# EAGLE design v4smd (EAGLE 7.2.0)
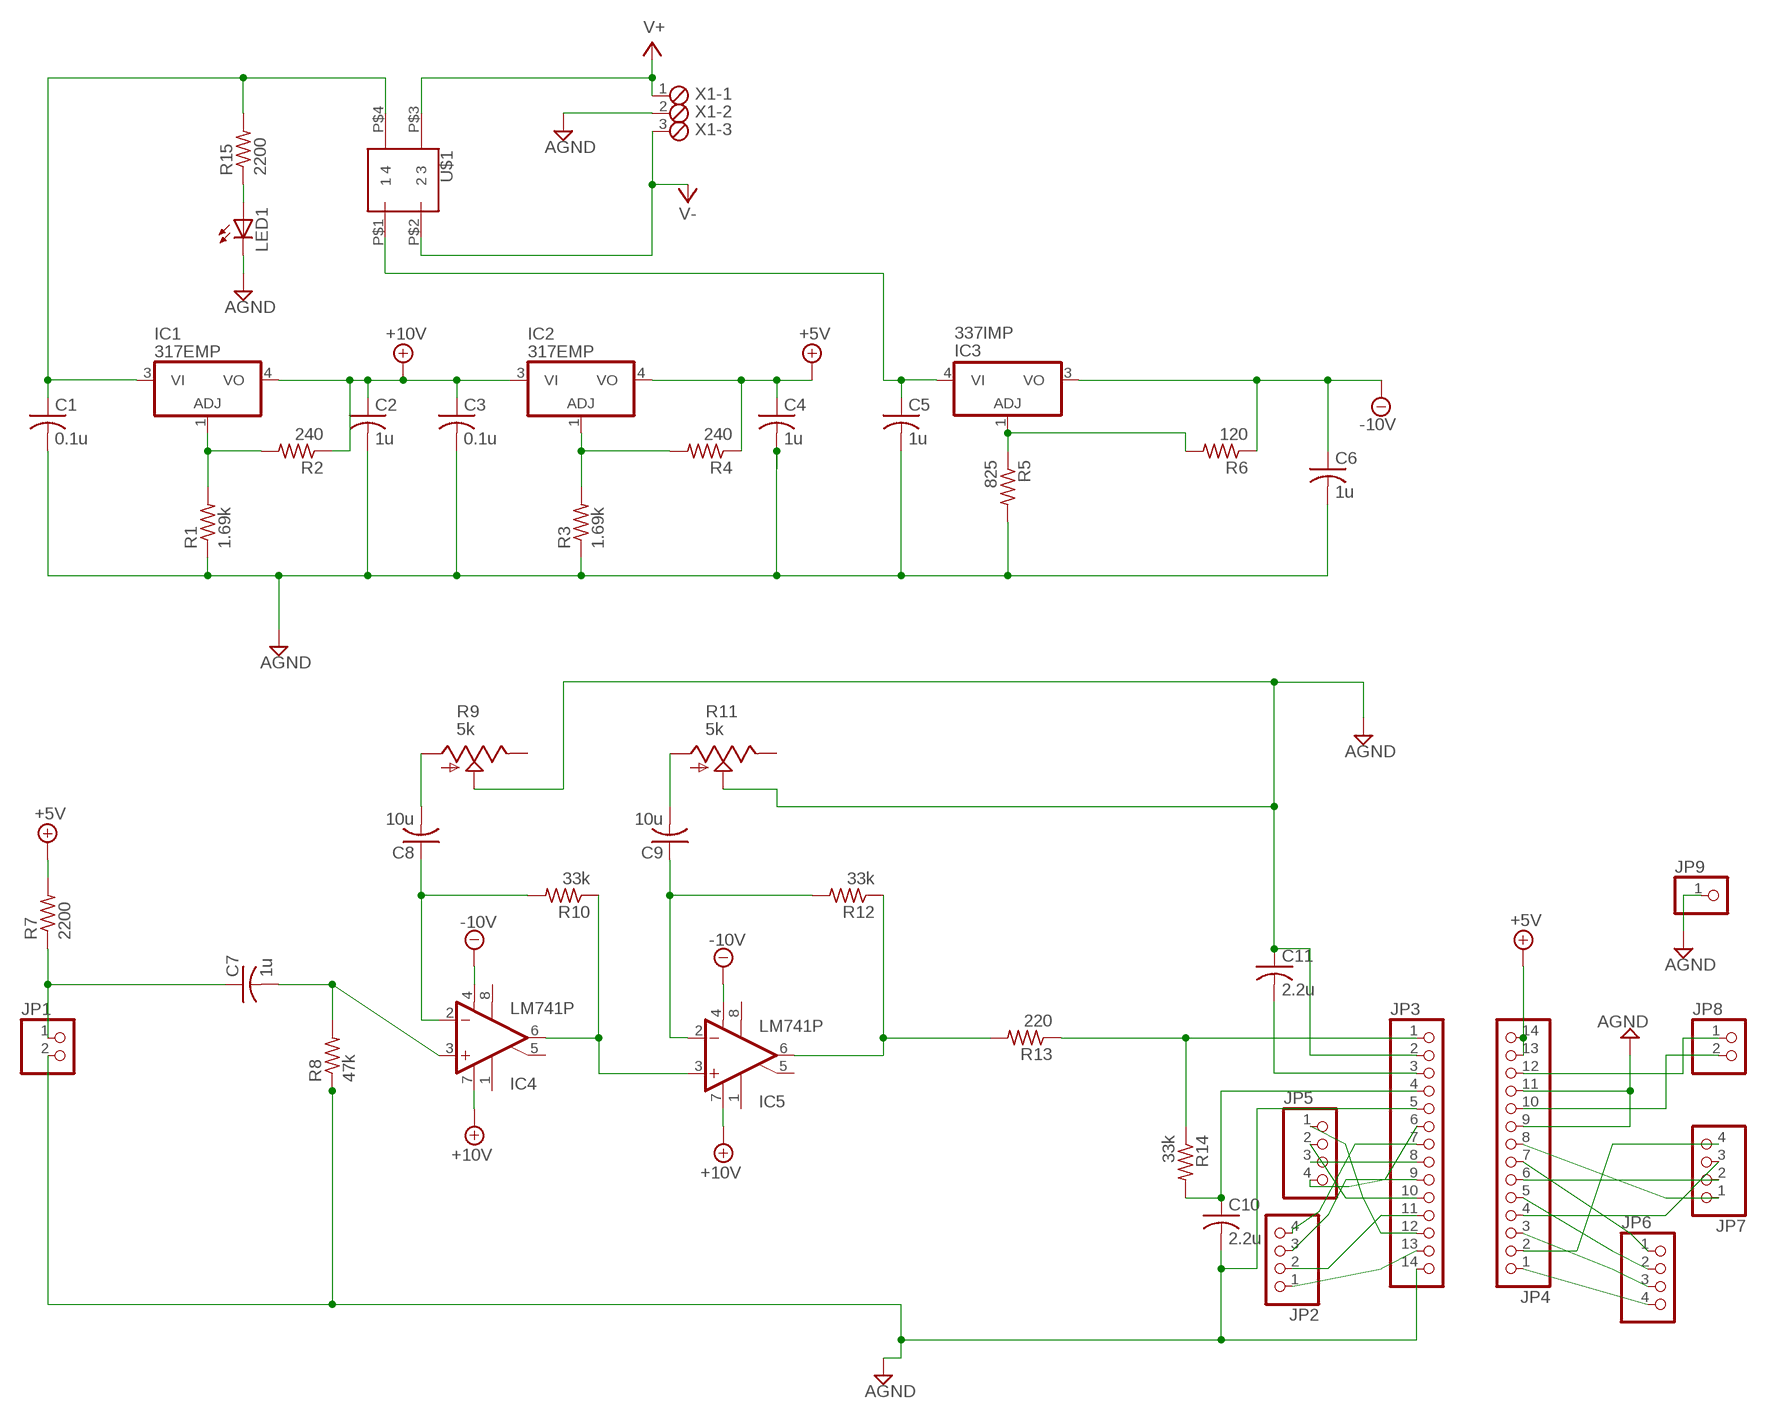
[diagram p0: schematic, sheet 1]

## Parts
C1  0.1u  C-USC1206  [C1206]
C2  1u  C-USC1206  [C1206]
C3  0.1u  C-USC1206  [C1206]
C4  1u  C-USC1206  [C1206]
C5  1u  C-USC1206  [C1206]
C6  1u  C-USC1206  [C1206]
C7  1u  C-USC1206  [C1206]
C8  10u  C-USC1206  [C1206]
C9  10u  C-USC1206  [C1206]
C10  2.2u  C-USC1206  [C1206]
C11  2.2u  C-USC1206  [C1206]
IC1  317EMP  [SOT223]
IC2  317EMP  [SOT223]
IC3  337IMP  [SOT223]
IC4  LM741P  [DIL08]
IC5  LM741P  [DIL08]
JP1  PINHD-1X2  [1X02]
JP2  PINHD-1X4/90  [1X04/90]
JP3  PINHD-1X14  [1X14]
JP4  PINHD-1X14  [1X14]
JP5  PINHD-1X4/90  [1X04/90]
JP6  PINHD-1X4/90  [1X04/90]
JP7  PINHD-1X4/90  [1X04/90]
JP8  PINHD-1X2  [1X02]
JP9  PINHD-1X1  [1X01]
LED1  LED3MM  [LED3MM]
R1  1.69k  R-US_R2512  [R2512]
R2  240  R-US_R2512  [R2512]
R3  1.69k  R-US_R2512  [R2512]
R4  240  R-US_R2512  [R2512]
R5  825  R-US_R2512  [R2512]
R6  120  R-US_R2512  [R2512]
R7  2200  R-US_R2512  [R2512]
R8  47k  R-US_R2512  [R2512]
R9  5k  TRIM_US-B64Y  [B64Y]
R10  33k  R-US_R2512  [R2512]
R11  5k  TRIM_US-B64Y  [B64Y]
R12  33k  R-US_R2512  [R2512]
R13  220  R-US_R2512  [R2512]
R14  33k  R-US_R2512  [R2512]
R15  2200  R-US_R2512  [R2512]
U$1  S201031MS02Q  [DPST_FOOTPRINT]
X1  MPT3  [3POL254]

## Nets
+5V: C4.1 IC2.4(VO) JP4.13 JP4.14 R4.1 R7.2
+10V: C2.1 C3.1 IC1.4(VO) IC2.3(VI) IC4.7(V+) IC5.7(V+) R2.1
-10V: C6.1 IC3.3(VO) IC4.4(V-) IC5.4(V-) R6.1
AGND: C1.2 C2.2 C3.2 C4.2 C5.2 C6.2 C10.2 C11.1 JP1.2 JP3.2 JP3.5 JP3.14 JP4.9 JP4.11 JP9.1 LED1.K(C) R1.1 R3.1 R5.2 R8.1 R9.S R11.S X1.2
N$1: IC4.6(OUT) IC5.3(+IN) R10.1
N$2: C7.1 JP1.1 R7.1
N$3: C7.2 IC4.3(+IN) R8.2
N$4: C8.1 IC4.2(-IN) R10.2
N$5: IC5.6(OUT) R12.1 R13.2
N$6: C9.1 IC5.2(-IN) R12.2
N$7: JP3.1 R13.1 R14.1
N$8: IC1.1(ADJ) R1.2 R2.2
N$9: IC2.1(ADJ) R3.2 R4.2
N$10: IC3.1(ADJ) R5.1 R6.2
N$11: C8.2 R9.A
N$12: JP4.2 JP7.4
N$13: JP4.3 JP6.3
N$14: C9.2 R11.A
N$15: C11.2 JP3.3
N$16: C10.1 JP3.4 R14.2
N$17: JP4.4 JP7.3
N$18: JP4.5 JP6.2
N$19: JP3.10 JP5.2
N$20: JP2.2 JP3.11
N$21: JP3.12 JP5.1
N$22: JP2.1 JP3.13
N$23: JP4.1 JP6.4
N$24: JP4.6 JP7.2
N$25: JP4.7 JP6.1
N$26: JP4.8 JP7.1
N$27: JP2.3 JP3.9
N$28: JP3.8 JP5.3
N$29: JP2.4 JP3.7
N$30: JP3.6 JP5.4
N$31: JP4.12 JP8.1
N$32: JP4.10 JP8.2
N$43: C1.1 IC1.3(VI) R15.2 U$1.P$4
N$44: C5.1 IC3.4(VI) U$1.P$1
N$45: LED1.A R15.1
V+: U$1.P$3 X1.1
V-: U$1.P$2 X1.3
Unconnected: IC4.1(ON1) IC4.5(ON2) IC4.8(OPT) IC5.1(ON1) IC5.5(ON2) IC5.8(OPT) R9.E R11.E

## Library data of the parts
C1-C11 = rcl:C-US: CAPACITOR, American symbol
IC1 IC2 = linear:*317: Positive VOLTAGE REGULATOR
IC3 = linear:*337: Negative VOLTAGE REGULATOR
IC4 IC5 = linear:*741: OP AMP
JP1 JP8 = pinhead:PINHD-1X2: PIN HEADER
JP2 JP5-JP7 = pinhead:PINHD-1X4: PIN HEADER
JP3 JP4 = pinhead:PINHD-1X14: PIN HEADER
JP9 = pinhead:PINHD-1X1: PIN HEADER
LED1 = led:LED: LED
R1-R8 R10 R12-R15 = rcl:R-US_: RESISTOR, American symbol
R9 R11 = pot:TRIM_US-: POTENTIOMETER
U$1 = mylib:S201031MS02Q
X1 = con-phoenix-254:MPT3: PHOENIX CONNECTOR; OC_FARNELL: unknown; OC_NEWARK: unknown

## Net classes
0 default: clearance 0.205 mm

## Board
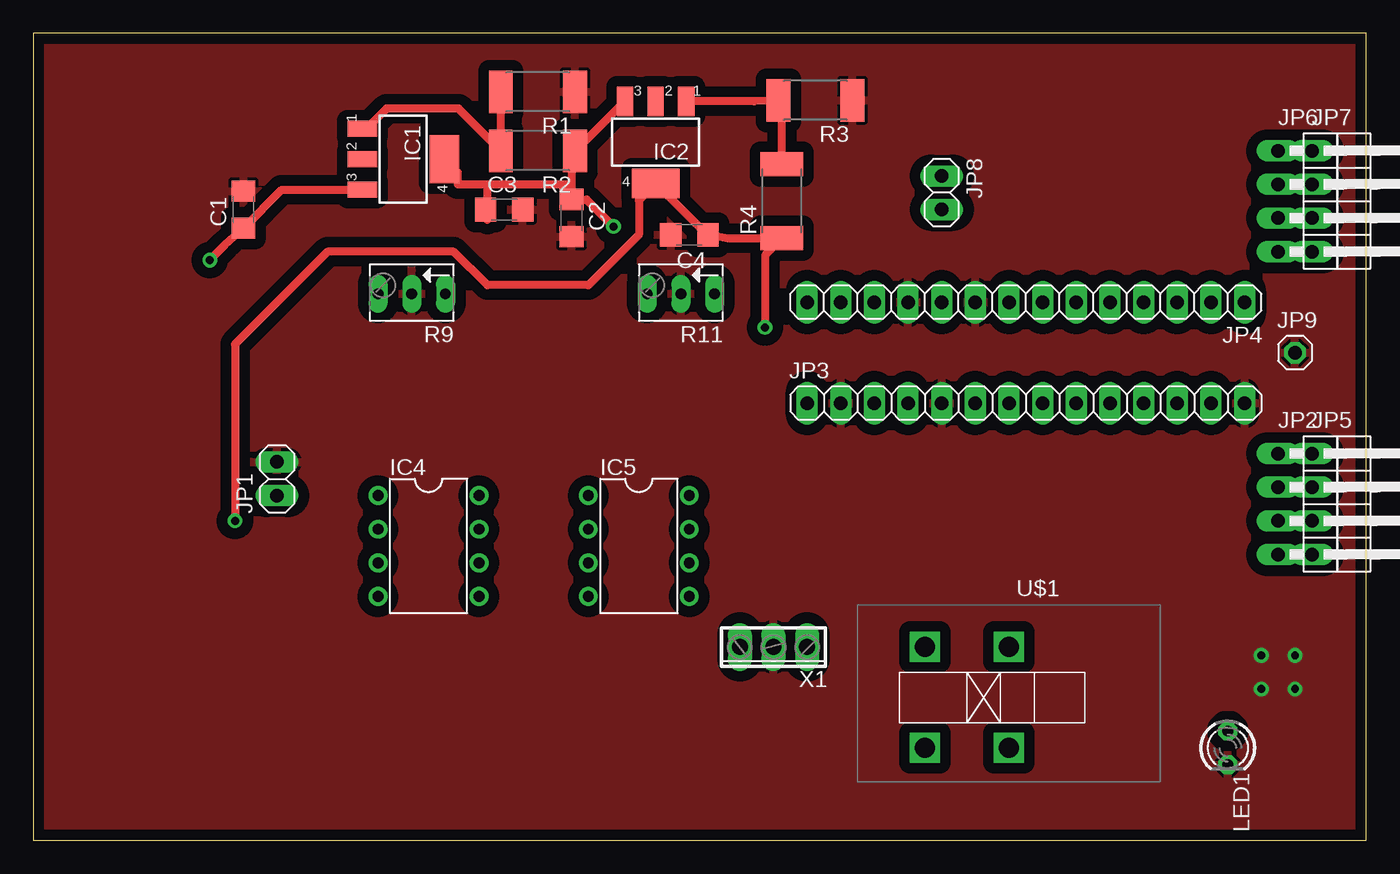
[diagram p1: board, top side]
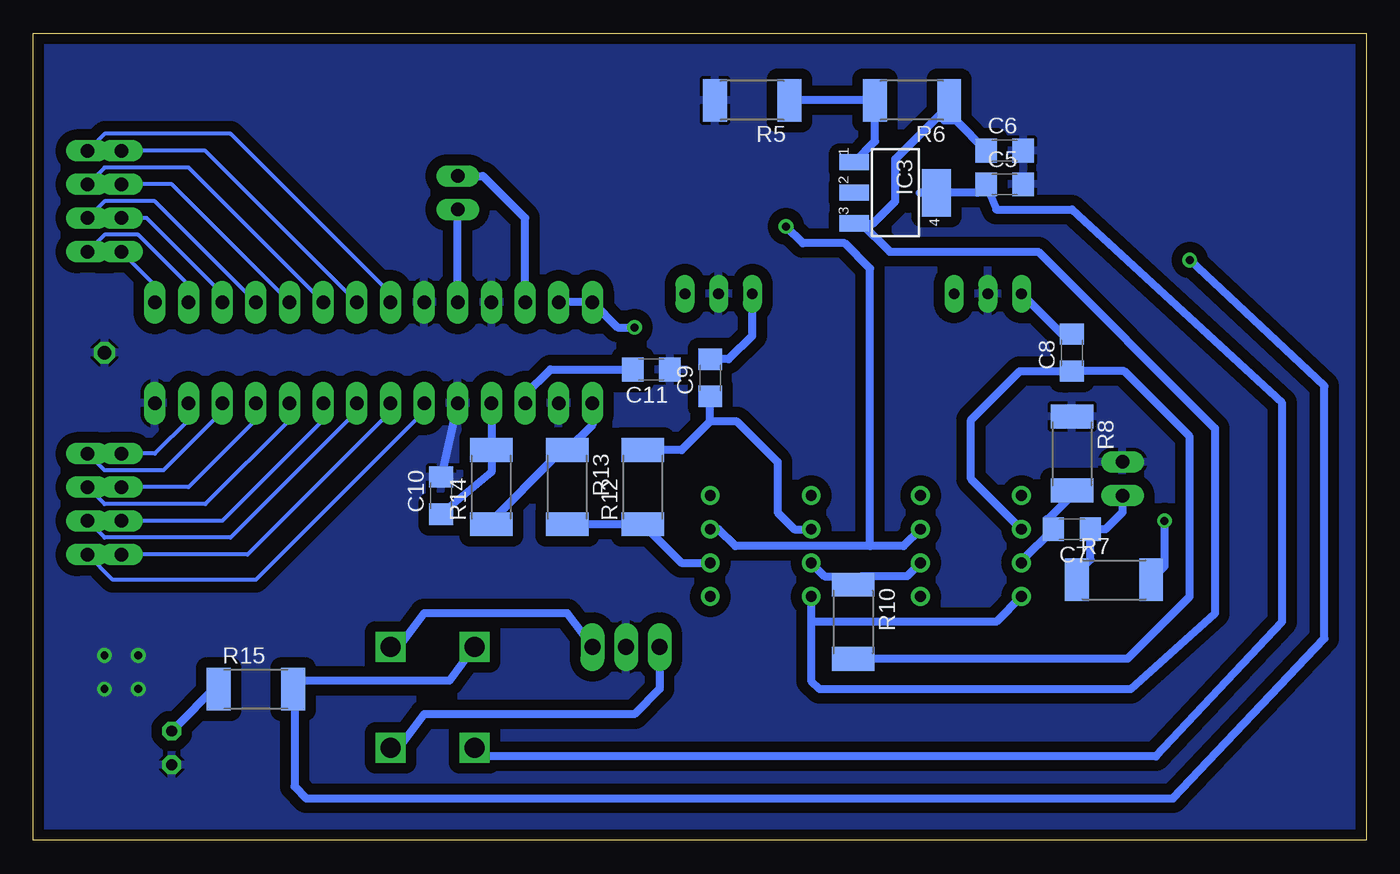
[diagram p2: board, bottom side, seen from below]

Size 100.64 x 60.95 mm. Coordinates in mm from the lower left corner, seen from the top.
Outline: 0,0 100.64,0 100.64,60.95 0,60.95 0,0
Copper layers (1*16): Top 0.035mm / dielectric 1.5mm / Bottom 0.035mm
Design rules "SparkFun": minimum track width 8mil, minimum drill 20mil, track to track 8mil, track to pad 8mil, pad to pad 8mil, via to via 8mil, smd to smd 8mil, copper to edge 10mil, drill to drill 8mil, minimum pad ring 12mil, minimum via ring 10mil, stop-mask expansion 4mil, vias tented up to drill 25mil, thermal gap 10mil

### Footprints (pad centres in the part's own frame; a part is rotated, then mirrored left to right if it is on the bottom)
C1206 = smd 1.6 x 1.8: 1 -1.4,0; 2 1.4,0
SOT223 = smd 1.219 x 2.235: 1 -2.311,-3.099; 2 0,-3.099; 3 2.311,-3.099 | smd 3.6 x 2.2: 4 0,3.099
DIL08 = drill 0.813 pad 1.27: 1 -3.81,-3.81; 2 -1.27,-3.81; 3 1.27,-3.81; 4 3.81,-3.81; 5 3.81,3.81; 6 1.27,3.81; 7 -1.27,3.81; 8 -3.81,3.81
1X02 = drill 1.016 long: 1 -1.27,0; 2 1.27,0
1X04/90 = drill 1.016 long: 1 -3.81,-3.81; 2 -1.27,-3.81; 3 1.27,-3.81; 4 3.81,-3.81
1X14 = drill 1.016 long: 1 -16.51,0; 2 -13.97,0; 3 -11.43,0; 4 -8.89,0; 5 -6.35,0; 6 -3.81,0; 7 -1.27,0; 8 1.27,0; 9 3.81,0; 10 6.35,0; 11 8.89,0; 12 11.43,0; 13 13.97,0; 14 16.51,0
1X01 = drill 1.016 octagon: 1 0,0
LED3MM = drill 0.813 octagon: A -1.27,0; K 1.27,0
R2512 = smd 1.8 x 3.2: 1 -2.8,0; 2 2.8,0
B64Y = drill 0.813 long: A 2.54,0; E -2.54,0; S 0,0
DPST_FOOTPRINT = drill 1.5 square: P$1 0,5.08; P$2 -6.35,5.08; P$3 -6.35,-2.54; P$4 0,-2.54
3POL254 = drill 1.2 long: 1 -2.54,0; 2 0,0; 3 2.54,0

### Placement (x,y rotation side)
C1  15.88,47.62 90 top
C2  40.64,46.99 270 top
C3  35.56,47.62 0 top
C4  49.53,45.72 180 top
C5  27.3,49.53 0 bottom
C6  27.3,52.07 0 bottom
C7  22.23,23.5 180 bottom
C8  22.23,36.83 90 bottom
C9  49.53,34.92 90 bottom
C10  69.85,26.04 90 bottom
C11  53.98,35.56 180 bottom
IC1  27.94,51.44 270 top
IC2  46.99,52.7 180 top
IC3  35.56,48.9 270 bottom
IC4  29.84,22.23 270 top
IC5  45.72,22.23 270 top
JP1  18.41,27.3 90 top
JP2  97.79,25.4 270 top
JP3  74.93,33.02 0 top
JP4  74.93,40.64 180 top
JP5  100.33,25.4 270 top
JP6  97.79,48.26 270 top
JP7  100.33,48.26 270 top
JP8  68.58,48.9 270 top
JP9  95.25,36.83 0 top
LED1  90.17,6.99 270 top
R1  38.1,56.52 180 top
R2  38.1,52.07 180 top
R3  59.05,55.88 180 top
R4  56.52,48.26 90 top
R5  46.35,55.88 180 bottom
R6  34.29,55.88 180 bottom
R7  19.05,19.68 0 bottom
R8  22.23,29.21 270 bottom
R9  28.57,41.27 180 top
R10  38.73,16.51 270 bottom
R11  48.9,41.27 180 top
R12  54.61,26.67 90 bottom
R13  60.33,26.67 270 bottom
R14  66.04,26.67 90 bottom
R15  83.82,11.43 0 bottom
U$1  67.31,12.06 180 top
X1  55.88,14.61 180 top

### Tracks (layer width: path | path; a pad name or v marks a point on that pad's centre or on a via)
+5V  (via drill 0.6)
  Top 0.61: v55.24,38.73 55.24,44.19 R4.1 52.46,45.46 C4.1 50.88,45.72 IC2.4 45.72,48.34 45.72,45.72 41.91,41.91 34.29,41.91 31.75,44.45 22.23,44.45 15.24,37.47 v15.24,24.13
  Bottom 0.61: JP4.13 JP4.14 56.52,38.73 v55.24,38.73 | v15.24,24.13 15.24,20.7 R7.2
+10V  (via drill 0.6)
  Top 0.61: IC2.3 40.95,52.07 R2.1 40.64,51.81 40.64,49.53 | 40.64,49.53 C2.1 41.78,48.39 v43.81,46.35 | 34.29,49.53 32.05,49.53 32.05,50.42 IC1.4 | 34.29,49.53 40.64,49.53 | C3.1 34.29,46.86 34.29,49.53
  Bottom 0.61: 37.47,22.23 37.47,43.18 39.37,45.09 42.55,45.09 v43.81,46.35 | IC4.7 34.92,22.23 37.47,22.23 | 37.47,22.23 47.62,22.23 48.9,23.5 IC5.7
-10V
  Bottom 0.61: R6.1 31.62,55.38 | 31.62,55.38 31.88,54.37 31,54.37 C6.1 | IC3.3 38.1,46.58 | 38.1,46.58 37.24,46.58 35.56,48.26 35.56,51.44 31.62,55.38 | 41.91,17.78 IC5.4 41.91,16.51 | 41.91,16.51 41.91,12.06 41.27,11.43 17.78,11.43 11.43,17.14 11.43,31.11 24.77,44.45 35.97,44.45 38.1,46.58 | IC4.4 27.94,16.51 41.91,16.51
AGND  (via drill 0.6)
  Bottom 0.61: JP3.5 C10.2
  other vias: 92.71,13.97 95.25,13.97 92.71,11.43 95.25,11.43
  pour Top (isolate 0.813): 0,60.96 0,0 102.23,0 102.87,60.96
  pour Bottom (isolate 0.813): -0.64,61.59 -0.64,0 103.5,0 103.5,61.59
N$1
  Bottom 0.61: R10.1 38.1,19.95 | IC4.6 34.66,19.95 38.1,19.95 | IC5.3 40.9,19.95 38.1,19.95
N$2
  Bottom 0.61: R7.1 22.09,19.93 20.82,21.2 C7.1 19.68,23.5 18.41,24.77 JP1.1
N$3
  Bottom 0.61: R8.2 22.23,26.04 24,24.26 24.13,24.26 C7.2 26.04,21.09 IC4.3
N$4
  Bottom 0.61: 39.37,13.97 R10.2 | 38.73,13.97 R10.2 | C8.1 18.29,35.43 13.34,30.48 13.34,18.41 18.04,13.71 R10.2 | C8.1 22.73,34.92 | C8.1 26.16,35.43 29.84,31.75 29.84,27.3 IC4.2
N$5
  Bottom 0.61: R13.2 R12.1 51.7,20.95 IC5.6
N$6
  Bottom 0.61: R12.2 51.68,29.47 49.53,31.62 | 49.53,31.62 C9.1 | 49.53,31.62 47.49,31.62 44.45,28.57 44.45,24.77 43.18,23.5 IC5.2
N$7
  Bottom 0.61: JP3.1 58.42,31.38 R13.1 60.7,29.47 66.67,23.5 66.42,23.5 R14.1
N$8
  Top 0.61: R1.2 R2.2 32.12,55.24 26.67,55.24 25.17,53.75 IC1.1
N$9
  Top 0.61: IC2.1 54.43,55.8 R3.2 56.52,55.62 R4.2
N$10
  Bottom 0.61: R5.1 R6.2 37.09,52.77 IC3.1
N$11
  Bottom 0.61: C8.2 22.99,38.23 R9.A
N$12
  Bottom 0.305: JP4.2 88.9,41.91 92.71,45.72 95.25,45.72 JP7.4
N$13
  Bottom 0.305: JP4.3 86.36,41.27 92.08,46.99 JP6.3
N$14
  Bottom 0.61: R11.A 46.35,38.1 48.13,36.33 C9.2
N$15
  Bottom 0.61: JP3.3 63.5,33.66 61.59,35.56 C11.2
N$16
  Bottom 0.61: JP3.4 R14.2 66.04,27.81 C10.1
N$17
  Bottom 0.305: JP4.4 91.44,48.26 95.25,48.26 JP7.3
N$18
  Bottom 0.305: JP4.5 90.17,49.53 JP6.2
N$19
  Bottom 0.305: 81.28,31.75 87.63,25.4 95.25,25.4 JP5.2
  Bottom 0.61: JP3.10 81.28,31.75
N$20
  Bottom 0.305: 83.82,31.75 88.9,26.67 JP2.2
  Bottom 0.61: JP3.11 83.82,31.75
N$21
  Bottom 0.305: JP3.12 86.36,32.38 90.81,27.94 95.25,27.94 JP5.1
N$22
  Bottom 0.305: JP3.13 88.9,31.75 91.44,29.21 JP2.1
N$23
  Bottom 0.305: JP4.1 91.44,41.91 JP6.4
N$24
  Bottom 0.305: JP4.6 88.9,50.8 95.25,50.8 JP7.2
N$25
  Bottom 0.305: JP4.7 87.63,52.07 JP6.1
N$26
  Bottom 0.305: JP4.8 73.66,41.27 85.72,53.34 95.25,53.34 JP7.1
N$27
  Bottom 0.305: JP3.9 78.74,31.75 86.36,24.13 JP2.3
N$28
  Bottom 0.305: JP3.8 76.2,32.38 85.72,22.86 95.25,22.86 JP5.3
N$29
  Bottom 0.305: JP3.7 73.66,32.38 84.45,21.59 JP2.4
N$30
  Bottom 0.305: JP3.6 71.12,32.38 83.82,19.68 94.61,19.68 JP5.4
N$31
  Bottom 0.61: JP4.12 63.5,46.99 66.67,50.16 JP8.1
N$32
  Bottom 0.61: JP4.10 JP8.2
N$43  (via drill 0.6)
  Top 0.61: v13.34,43.81 14.47,44.95 C1.1 18.77,49.12 IC1.3
  Bottom 0.61: v13.34,43.81 3.17,34.29 3.17,15.24 14.61,3.17 80.01,3.17 80.91,4.07 80.91,11.05 81.28,11.43 R15.2 81.02,12.44 81.28,12.06 69.22,12.06 U$1.P$4
N$44
  Bottom 0.61: 33.73,48.9 IC3.4 29.34,48.9 C5.1 27.94,47.62 22.23,47.62 6.35,33.02 6.35,16.51 15.88,6.35 67.31,6.35 U$1.P$1
N$45
  Bottom 0.61: R15.1 86.62,11.8 LED1.A
V+
  Bottom 0.61: X1.1 60.33,17.14 71.12,17.14 73.03,14.61 U$1.P$3
V-
  Bottom 0.61: U$1.P$2 73.03,6.99 71.12,9.53 55.24,9.53 53.34,11.43 X1.3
